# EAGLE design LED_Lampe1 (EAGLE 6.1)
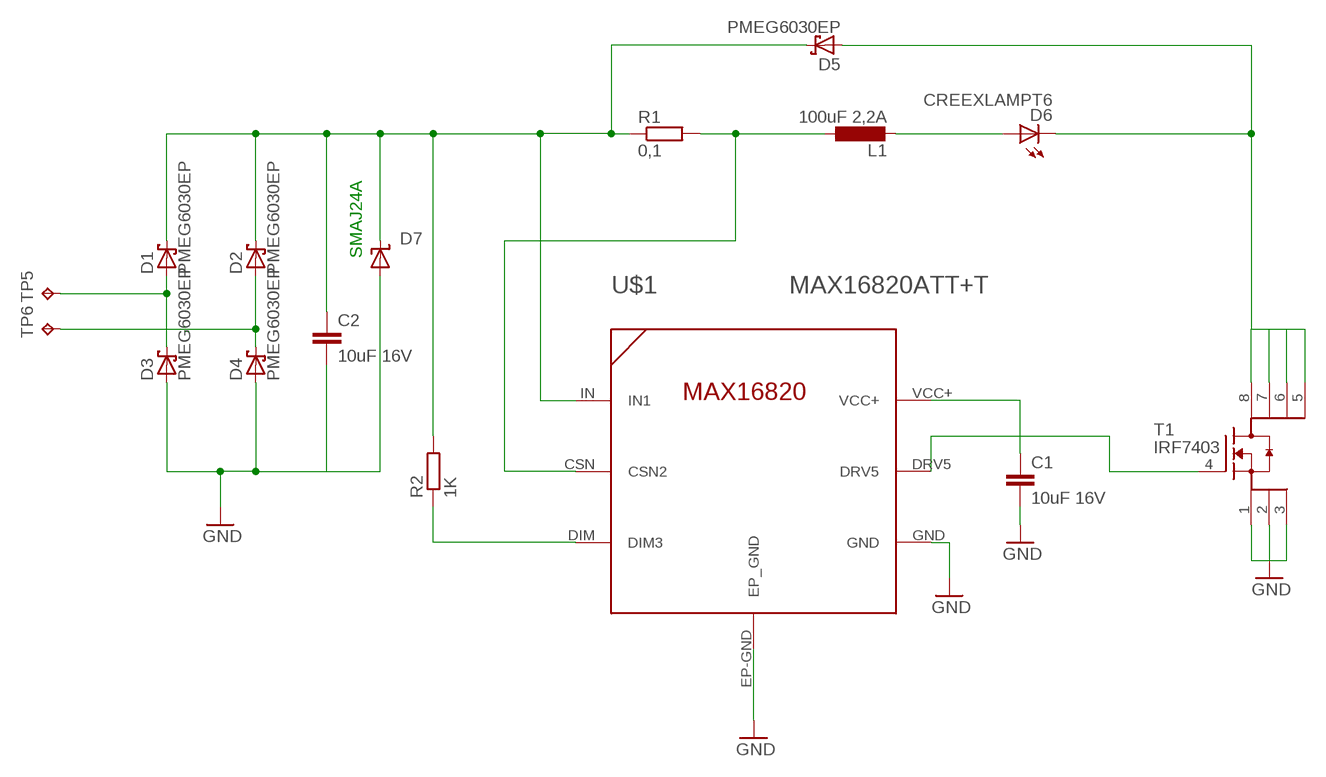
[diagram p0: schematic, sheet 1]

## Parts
C1  10uF 16V  C-EUC1210  [C1210]
C2  10uF 16V  C-EUC1210  [C1210]
D1  PMEG6030EP  [SOD128]
D2  PMEG6030EP  [SOD128]
D3  PMEG6030EP  [SOD128]
D4  PMEG6030EP  [SOD128]
D5  PMEG6030EP  [SOD128]
D6  CREEXLAMPT6  [CREEXLAMPXMLT6]
D7  SUPPRESSOR-SMBJ  [SMBJ]
L1  100uF 2,2A  L-EU  [L12-7]
R1  0,1  R-EU_R2512  [R2512]
R2  1K  R-EU_R1206  [R1206]
T1  IRF7403  [SO8]
TP5  TPTP20SQ  [TP20SQ]
TP6  TPTP20SQ  [TP20SQ]
U$1  MAX16820ATT+T  [TDFN6]

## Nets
GND: C1.2 C2.2 D3.2(A) D4.2(A) D7.A T1.1(S) T1.2(S) T1.3(S) U$1.EP-GND(EP_GND) U$1.GND
N$1: D6.A+(A) L1.P$2
N$4: T1.4(G) U$1.DRV5
N$5: D5.2(A) D6.K-(C) T1.5(D) T1.6(D) T1.7(D) T1.8(D)
N$6: L1.P$1 R1.2 U$1.CSN(CSN2)
N$7: C2.1 D1.1(K) D2.1(K) D5.1(K) D7.C R1.1 R2.2 U$1.IN(IN1)
N$9: R2.1 U$1.DIM(DIM3)
N$11: D1.2(A) D3.1(K) TP5.TP
N$12: D2.2(A) D4.1(K) TP6.TP
VCC+: C1.1 U$1.VCC+

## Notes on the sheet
- SMAJ24A

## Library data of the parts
C1 C2 = rcl:C-EU: CAPACITOR, European symbol
D1-D5 = nxp_60_1_1:PMEG6030: 60V 3A low VF dual MEGA Schottky barrier rectifier
D6 = led:CREEXLAMPT6
D7 = Diode_mod:SUPPRESSOR-: Suppressor diode
L1 = rcl:L-EU: INDUCTOR, European symbol
R1 R2 = rcl:R-EU_: RESISTOR, European symbol
T1 = 1_USER:IRF7403
TP5 TP6 = testpad:TP: Test pad
U$1 = maxim_mod:MAX16820ATT+T

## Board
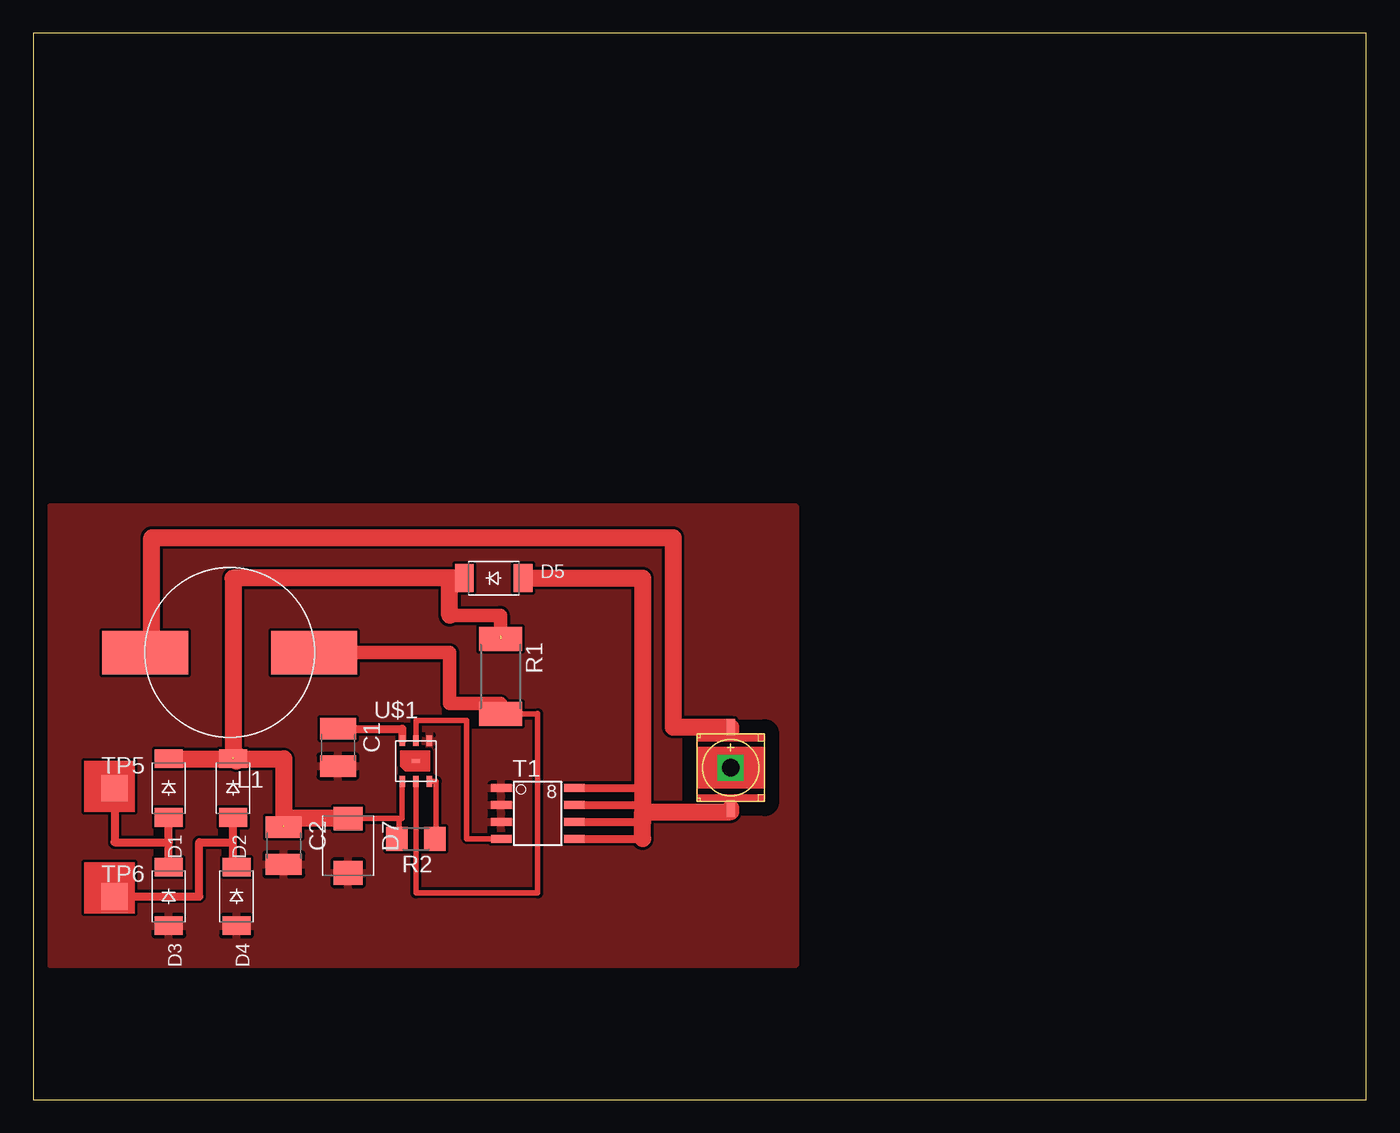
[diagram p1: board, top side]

Size 100 x 80 mm. Coordinates in mm from the lower left corner, seen from the top.
Outline: 0,0 100,0 100,80 0,80 0,0
Copper layers (1*16): Top 0.035mm / dielectric 1.5mm / Bottom 0.035mm
Design rules: minimum track width 10mil, minimum drill 24mil, track to track 8mil, track to pad 8mil, pad to pad 8mil, via to via 8mil, smd to smd 8mil, copper to edge 40mil, drill to drill 8mil, minimum pad ring 10mil, minimum via ring 8mil, stop-mask expansion 4mil, vias tented up to drill 0mil, thermal gap 10mil
tKeepout: area 47,20.3 to 55.9,29.2

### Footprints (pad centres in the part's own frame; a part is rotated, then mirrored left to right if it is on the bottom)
C1210 = smd 1.6 x 2.7: 1 -1.4,0; 2 1.4,0
SOD128 = smd 1.4 x 2.1: 1 -2.2,0; 2 2.2,0
CREEXLAMPXMLT6 = smd 1.27 x 0.66: A+ 3.048,0; K- -3.048,0
SMBJ = smd 1.78 x 2.16: A 2.04,0; C -2.03,0
L12-7 = smd 6.452 x 3.251: P$1 -6.35,0; P$2 6.35,0
R2512 = smd 1.8 x 3.2: 1 -2.8,0; 2 2.8,0
R1206 = smd 1.6 x 1.803: 1 -1.422,0; 2 1.422,0
SO8 = smd 0.61 x 1.524: 1 -1.27,-2.743; 2 0,-2.743; 3 1.27,-2.743; 4 2.54,-2.743; 5 2.54,2.743; 6 1.27,2.743; 7 0,2.743; 8 -1.27,2.743
TP20SQ = smd 2 x 2: TP 0,0
TDFN6 = smd 0.406 x 0.813: CSN 0,-1.524; DIM 1.016,-1.524; DRV5 0,1.524; GND 1.016,1.524; IN -1.016,-1.524; VCC+ -1.016,1.524 | smd 0.61 x 0.305: EP-GND 0,0

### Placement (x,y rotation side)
C1  22.86,26.42 270 top
C2  18.8,19.05 270 top
D1  10.16,23.37 270 top
D2  14.99,23.37 270 top
D3  10.16,15.24 270 top
D4  15.24,15.24 270 top
D5  34.54,39.12 0 top
D6  52.32,24.89 90 top
D7  23.62,19.05 270 top
L1  14.73,33.53 180 top
R1  35.05,31.75 270 top
R2  28.7,19.56 180 top
T1  37.85,22.1 270 top
TP5  6.1,23.37 0 top
TP6  6.1,15.24 0 top
U$1  28.7,25.4 0 top

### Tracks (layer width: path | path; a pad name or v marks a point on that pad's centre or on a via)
GND
  pour Top: 1.27,44.45 57.15,44.45 57.15,10.16 1.27,10.16
N$1
  Top 1.27: L1.P$2 8.89,33.53 8.89,42.16 48.01,42.16 48.01,27.94 D6.A+ 52.32,27.69
N$2  (via drill 1.3 pad 1.78)
  other vias: 52.32,24.89
N$4
  Top 0.406: T1.4 32.51,19.56 32.51,28.45 28.7,28.45 U$1.DRV5
N$5
  Top 0.61: T1.8 45.72,23.37 45.72,21.84 | T1.7 45.72,22.1 45.72,22.35 | T1.6 45.72,20.83 | T1.5 45.72,19.56
  Top 1.27: D5.2 45.72,39.12 45.72,23.37 45.72,22.35 45.72,21.84 45.72,21.59 | 45.72,21.59 52.32,21.59 D6.K- | 45.72,21.59 45.72,20.83 45.72,19.56
N$6
  Top 0.406: 37.85,28.95 37.85,15.49 28.7,15.49 U$1.CSN | R1.2 37.85,28.95 | 37.85,28.95 37.85,28.96
  Top 1.016: L1.P$1 31.24,33.53 31.24,29.72 35.05,29.72 R1.2
N$7  (3 unrouted)
  Top 0.406: 18.8,21.08 C2.1 | D7.C 27.43,21.08 | 27.43,21.08 27.69,21.08 U$1.IN | R2.2 27.43,19.56 27.43,21.08
  Top 1.016: 31.24,36.32 35.05,36.32 35.05,34.8
  Top 1.27: D1.1 D2.1 18.8,25.57 18.8,20.57 | D7.C 18.8,21.08 | D5.1 31.24,39.12 | 31.24,39.12 14.99,39.12 14.99,25.91 | 14.99,25.65 14.99,25.91 | 14.99,25.91 15.24,25.91 15.24,25.4 | 31.24,36.32 31.24,39.12
N$9
  Top 0.406: R2.1 30.23,19.56 30.23,23.88 U$1.DIM
N$11
  Top 0.61: D3.1 10.16,19.3 | 10.16,19.3 D1.2 | TP5.TP 6.1,19.3 10.16,19.3
N$12
  Top 0.406: D4.1 14.99,17.44
  Top 0.61: 14.99,17.44 14.99,19.3 | 14.99,19.3 D2.2 | TP6.TP 12.45,15.24 12.45,19.3 14.99,19.3
VCC+
  Top 0.61: C1.1 27.69,27.82 U$1.VCC+
(copper drawn outside any net)
  shapes: Top area x2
